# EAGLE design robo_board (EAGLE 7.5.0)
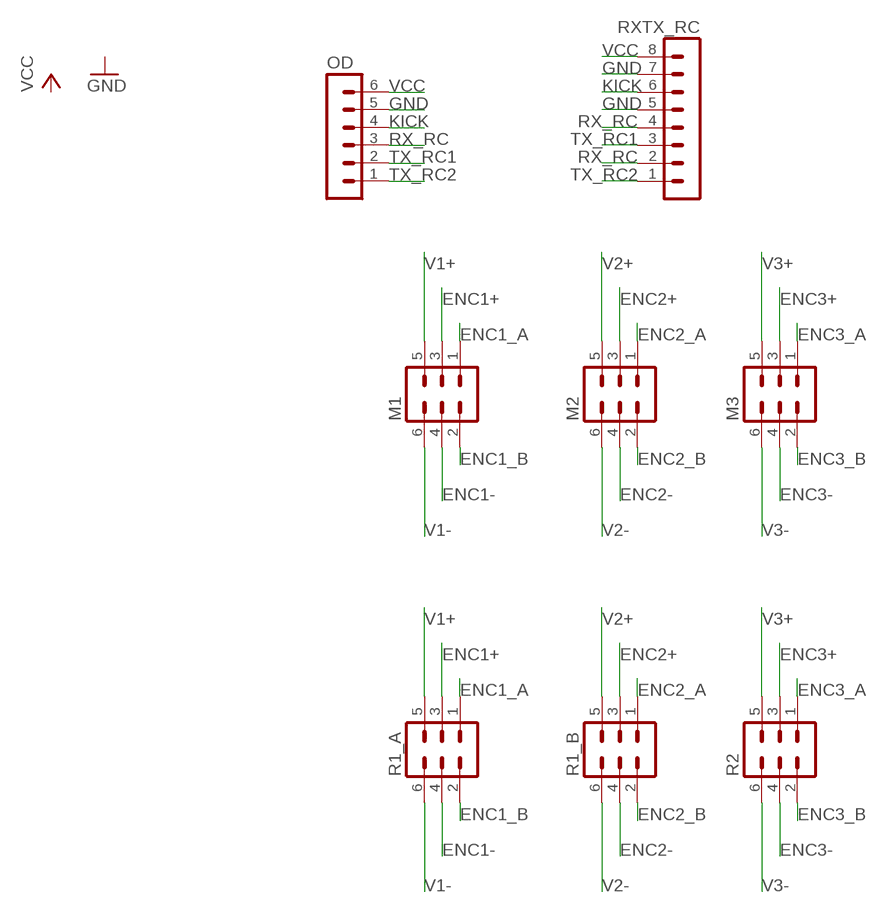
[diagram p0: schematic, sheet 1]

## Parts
M1  MA03-2  [MA03-2]
M2  MA03-2  [MA03-2]
M3  MA03-2  [MA03-2]
OD  MA06-1  [MA06-1]
R1_A  MA03-2  [MA03-2]
R1_B  MA03-2  [MA03-2]
R2  MA03-2  [MA03-2]
RXTX_RC  MA08-1  [MA08-1]

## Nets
ENC1+: M1.3 R1_A.3
ENC1-: M1.4 R1_A.4
ENC1_A: M1.1 R1_A.1
ENC1_B: M1.2 R1_A.2
ENC2+: M2.3 R1_B.3
ENC2-: M2.4 R1_B.4
ENC2_A: M2.1 R1_B.1
ENC2_B: M2.2 R1_B.2
ENC3+: M3.3 R2.3
ENC3-: M3.4 R2.4
ENC3_A: M3.1 R2.1
ENC3_B: M3.2 R2.2
GND: OD.5 RXTX_RC.5 RXTX_RC.7
KICK: OD.4 RXTX_RC.6
RX_RC: OD.3 RXTX_RC.2 RXTX_RC.4
TX_RC1: OD.2 RXTX_RC.3
TX_RC2: OD.1 RXTX_RC.1
V1+: M1.5 R1_A.5
V1-: M1.6 R1_A.6
V2+: M2.5 R1_B.5
V2-: M2.6 R1_B.6
V3+: M3.5 R2.5
V3-: M3.6 R2.6
VCC: OD.6 RXTX_RC.8

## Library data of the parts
M1-M3 R1_A R1_B R2 = con-lstb:MA03-2: PIN HEADER; OC_FARNELL: unknown; OC_NEWARK: unknown
OD = con-lstb:MA06-1: PIN HEADER; OC_FARNELL: unknown; OC_NEWARK: unknown
RXTX_RC = con-lstb:MA08-1: PIN HEADER; OC_FARNELL: unknown; OC_NEWARK: unknown

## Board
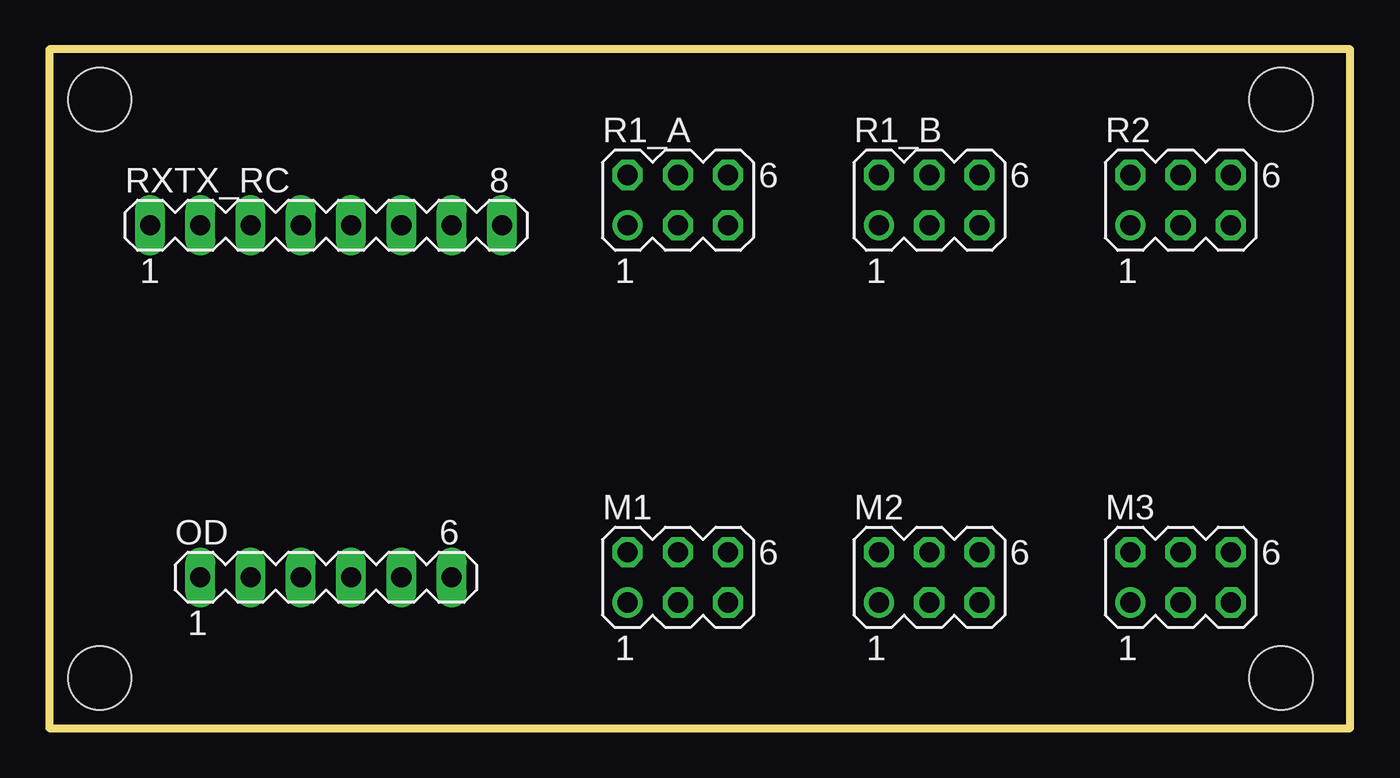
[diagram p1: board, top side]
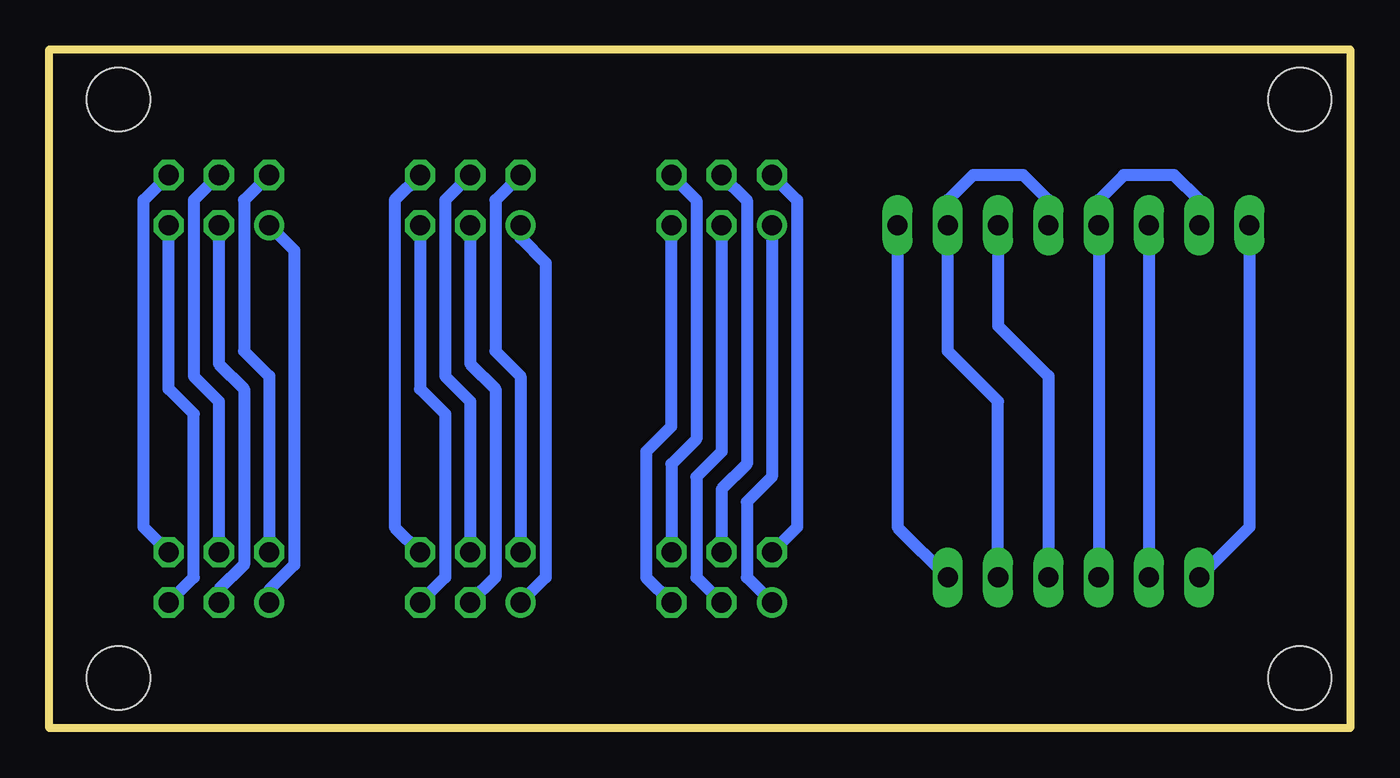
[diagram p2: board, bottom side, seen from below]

Size 65.71 x 34.28 mm. Coordinates in mm from the lower left corner, seen from the top.
Outline: 0,0 65.71,0 65.71,34.28 0,34.28 0,0
Copper layers (1*16): Top 0.035mm / dielectric 1.5mm / Bottom 0.035mm
Design rules "default *": minimum track width 24mil, minimum drill 32mil, track to track 8mil, track to pad 8mil, pad to pad 8mil, via to via 8mil, smd to smd 8mil, copper to edge 40mil, drill to drill 8mil, minimum pad ring 10mil, minimum via ring 8mil, stop-mask expansion 4mil, vias tented up to drill 0mil, thermal gap 10mil
Holes 3.2 mm at 2.54,31.75 2.54,2.54 62.23,2.54 62.23,31.75

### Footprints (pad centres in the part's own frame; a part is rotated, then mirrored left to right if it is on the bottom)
MA03-2 = drill 1.016: 1 -2.54,-1.27 | drill 1.016 octagon: 2 -2.54,1.27; 3 0,-1.27; 4 0,1.27; 5 2.54,-1.27; 6 2.54,1.27
MA06-1 = drill 1.016 long: 1 -6.35,0; 2 -3.81,0; 3 -1.27,0; 4 1.27,0; 5 3.81,0; 6 6.35,0
MA08-1 = drill 1.016 long: 1 -8.89,0; 2 -6.35,0; 3 -3.81,0; 4 -1.27,0; 5 1.27,0; 6 3.81,0; 7 6.35,0; 8 8.89,0

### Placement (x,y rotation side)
M1  31.75,7.62 0 top
M2  44.45,7.62 0 top
M3  57.15,7.62 0 top
OD  13.97,7.62 0 top
R1_A  31.75,26.67 0 top
R1_B  44.45,26.67 0 top
R2  57.15,26.67 0 top
RXTX_RC  13.97,25.4 0 top

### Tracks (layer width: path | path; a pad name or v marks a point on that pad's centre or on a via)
ENC1+
  Bottom 0.61: R1_A.3 31.75,13.97 33.02,12.7 33.02,7.62 M1.3
ENC1-
  Bottom 0.61: R1_A.4 30.48,26.67 30.48,13.34 31.75,12.06 M1.4
ENC1_A
  Bottom 0.61: R1_A.1 29.21,12.7 30.48,11.43 30.48,7.62 M1.1
ENC1_B
  Bottom 0.61: R1_A.2 27.94,26.67 27.94,10.16 M1.2
ENC2+
  Bottom 0.61: R1_B.3 44.45,18.41 43.18,17.14 43.18,7.62 M2.3
ENC2-
  Bottom 0.61: R1_B.4 45.72,26.67 45.72,17.78 44.45,16.51 M2.4
ENC2_A
  Bottom 0.61: M2.1 40.64,7.62 40.64,23.5 41.91,24.77 R1_B.1
ENC2_B
  Bottom 0.61: R1_B.2 43.18,26.67 43.18,19.05 41.91,17.78 M2.2
ENC3+
  Bottom 0.61: M3.3 57.15,6.99 55.88,8.26 55.88,17.14 57.15,18.41 R2.3
ENC3-
  Bottom 0.61: M3.4 57.15,16.51 58.42,17.78 58.42,26.67 R2.4
ENC3_A
  Bottom 0.61: M3.1 54.61,6.99 53.34,8.26 53.34,24.13 R2.1
ENC3_B
  Bottom 0.61: M3.2 54.61,17.78 55.88,19.05 55.88,26.67 R2.2
GND
  Bottom 0.61: RXTX_RC.5 15.24,26.67 16.51,27.94 19.05,27.94 20.32,26.67 RXTX_RC.7 20.32,19.05 17.78,16.51 OD.5
KICK
  Bottom 0.61: RXTX_RC.6 17.78,20.32 15.24,17.78 OD.4
RX_RC
  Bottom 0.61: RXTX_RC.2 7.62,26.67 8.89,27.94 11.43,27.94 12.7,26.67 RXTX_RC.4 OD.3
TX_RC1
  Bottom 0.61: RXTX_RC.3 OD.2
TX_RC2
  Bottom 0.61: RXTX_RC.1 5.08,10.16 OD.1
V1+
  Bottom 0.61: R1_A.5 34.29,15.24 35.56,13.97 35.56,7.62 M1.5
V1-
  Bottom 0.61: R1_A.6 33.02,26.67 33.02,14.61 34.29,13.34 M1.6
V2+
  Bottom 0.61: R1_B.5 46.99,17.14 45.72,15.88 45.72,7.62 M2.5
V2-
  Bottom 0.61: R1_B.6 48.26,26.67 48.26,10.16 M2.6
V3+
  Bottom 0.61: M3.5 58.42,7.62 58.42,15.88 59.69,17.14 R2.5
V3-
  Bottom 0.61: M3.6 60.96,10.16 60.96,26.67 R2.6
VCC
  Bottom 0.61: RXTX_RC.8 22.86,10.16 OD.6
